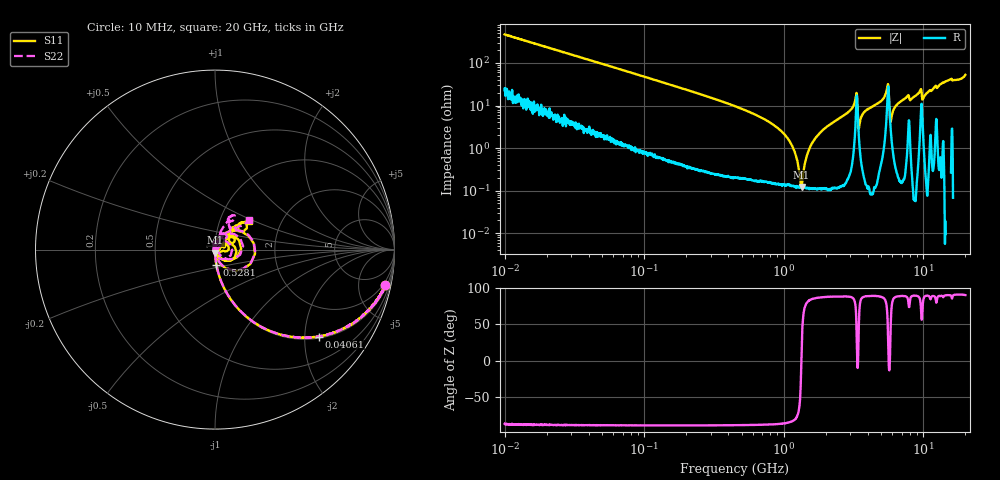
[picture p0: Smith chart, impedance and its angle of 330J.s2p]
!Keysight Technologies,P5008B,MY61100088,A.16.20.02
!Date: Tuesday, November 07, 2023 16:02:35
!Correction: S11(C  2-Port  )
!S21(C  2-Port  )
!S12(C  2-Port  )
!S22(C  2-Port  )
!S2P File: Measurements: S11, S21, S12, S22:Log Frequency Sweep
# Hz S  dB  R 50
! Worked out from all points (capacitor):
!   1601 points, 10 MHz to 20 GHz, reference 50 ohm
!   read as one part in series: C = 33.8 pF near 10.39 MHz
!   lowest |Z| = 122 mohm at 1.34 GHz (marker M1)
!   series resonance near 1.337 GHz, so ESL is about 420 pH
!   S11 on the Smith chart (normalised r, x): 10 MHz: 1.48, -9.37; 40.61 MHz: 1.05, -2.35; 528.1 MHz: 1.00, -0.17; 20 GHz: 1.37, +0.47
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1e7  -0.28 -11.9  -13.71 75.1  -13.71 75.1  -0.28 -11.9
3.555162e7  -2.02 -36.4  -4.54 52.3  -4.55 52.3  -2.02 -36.4
4.060948e7  -2.45 -40.0  -3.85 48.8  -3.86 48.8  -2.45 -40.0
1.263918e8  -9.04 -68.6  -0.63 20.5  -0.63 20.5  -9.04 -68.6
4.472136e8  -19.85 -83.7  -0.06 5.2  -0.06 5.2  -19.84 -83.6
5.281108e8  -21.47 -84.7  -0.05 4.0  -0.05 4.0  -21.47 -84.6
1.339989e9  -35.58 -81.3  -0.01 -1.0  -0.01 -1.0  -35.60 -92.3
1.589917e9  -42.28 -69.0  -0.01 -1.9  -0.01 -1.9  -42.52 -96.0
1.859765e9  -50.08 10.4  -0.01 -2.8  -0.01 -2.8  -65.32 155.3
2.064654e9  -43.76 58.8  -0.01 -3.5  -0.01 -3.4  -45.73 92.2
3.257685e9  -20.90 61.1  -0.29 -10.1  -0.30 -10.1  -20.59 59.7
3.616581e9  -41.70 113.4  -0.03 -6.2  -0.03 -6.1  -36.97 20.9
3.846973e9  -32.92 98.7  -0.01 -7.4  -0.01 -7.4  -32.61 57.4
5.652411e9  -14.38 -35.3  -1.58 -5.1  -1.58 -5.1  -14.44 -33.8
6.186336e9  -33.74 -57.0  -0.02 -10.8  -0.02 -10.8  -38.19 -98.9
6.425969e9  -35.36 -22.7  0.00 -12.0  -0.00 -11.9  -44.52 176.1
7.588373e9  -25.66 26.2  -0.02 -16.3  -0.03 -16.3  -27.45 102.1
8.305168e9  -33.56 -5.2  0.01 -17.0  0.01 -17.0  -38.78 132.9
9.486728e9  -22.54 29.7  -0.22 -22.8  -0.22 -22.7  -24.25 53.0
1.038284e10  -33.17 -7.3  0.02 -21.2  0.01 -21.2  -39.37 130.8
1.361179e10  -15.50 48.1  -0.11 -30.3  -0.11 -30.2  -15.50 65.9
2e10  -12.17 40.6  -0.28 -50.7  -0.28 -50.6  -12.06 41.1
